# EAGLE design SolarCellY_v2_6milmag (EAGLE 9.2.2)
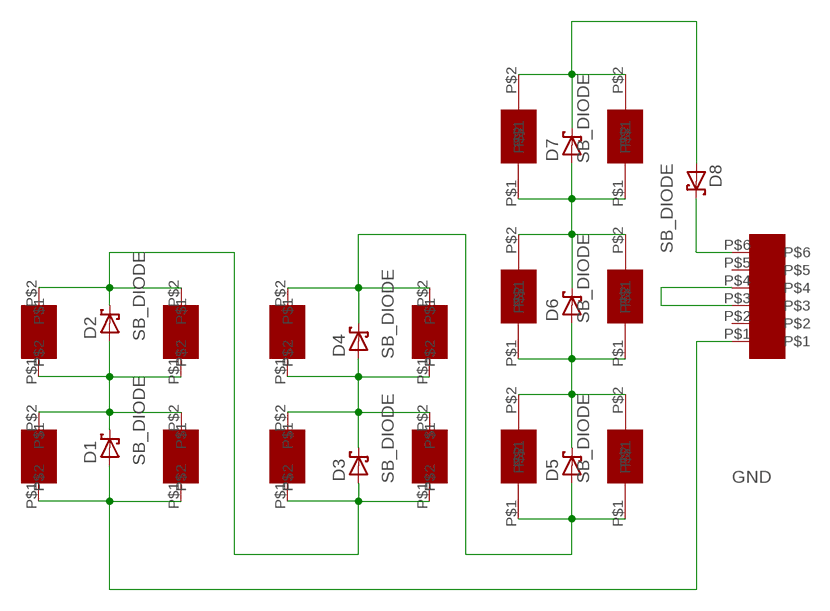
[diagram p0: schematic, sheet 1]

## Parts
11  SLMD121H04L  [SLMD121H04L]
12  SLMD121H04L  [SLMD121H04L]
13  SLMD121H04L  [SLMD121H04L]
14  SLMD121H04L  [SLMD121H04L]
21  SLMD121H04L  [SLMD121H04L]
22  SLMD121H04L  [SLMD121H04L]
23  SLMD121H04L  [SLMD121H04L]
24  SLMD121H04L  [SLMD121H04L]
D1  SB_DIODE  [SB_DIODE]
D2  SB_DIODE  [SB_DIODE]
D3  SB_DIODE  [SB_DIODE]
D4  SB_DIODE  [SB_DIODE]
D5  SB_DIODE  [SB_DIODE]
D6  SB_DIODE  [SB_DIODE]
D7  SB_DIODE  [SB_DIODE]
D8  SB_DIODE  [SB_DIODE]
U$1  M20-8760342  [M20-8760342]
U$2  KXOB22-04X3F  [KXOB22-04X3F]
U$3  KXOB22-04X3F  [KXOB22-04X3F]
U$4  KXOB22-04X3F  [KXOB22-04X3F]
U$5  KXOB22-04X3F  [KXOB22-04X3F]
U$6  KXOB22-04X3F  [KXOB22-04X3F]
U$7  KXOB22-04X3F  [KXOB22-04X3F]

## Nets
GND: 11.P$1 12.P$1 D1.POS U$1.P$1
N$1: U$1.P$3 U$1.P$4
N$2: 11.P$2 12.P$2 13.P$1 14.P$1 D1.NEG D2.POS
N$3: 13.P$2 14.P$2 21.P$1 22.P$1 D2.NEG D3.POS
N$4: 23.P$2 24.P$2 D4.NEG D5.POS U$2.P$1 U$3.P$1
N$5: 21.P$2 22.P$2 23.P$1 24.P$1 D3.NEG D4.POS
N$6: D5.NEG D6.POS U$2.P$2 U$3.P$2 U$4.P$1 U$5.P$1
N$8: D6.NEG D7.POS U$4.P$2 U$5.P$2 U$6.P$1 U$7.P$1
N$10: D7.NEG D8.POS U$6.P$2 U$7.P$2
N$14: D8.NEG U$1.P$6
Unconnected: U$1.P$2 U$1.P$5

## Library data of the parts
11-14 21-24 = Solar:SLMD121H04L
D1-D8 = Solar:SB_DIODE
U$1 = Solar:M20-8760342
U$2-U$7 = Solar:KXOB22-04X3F

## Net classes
1 power: width 0.254 mm

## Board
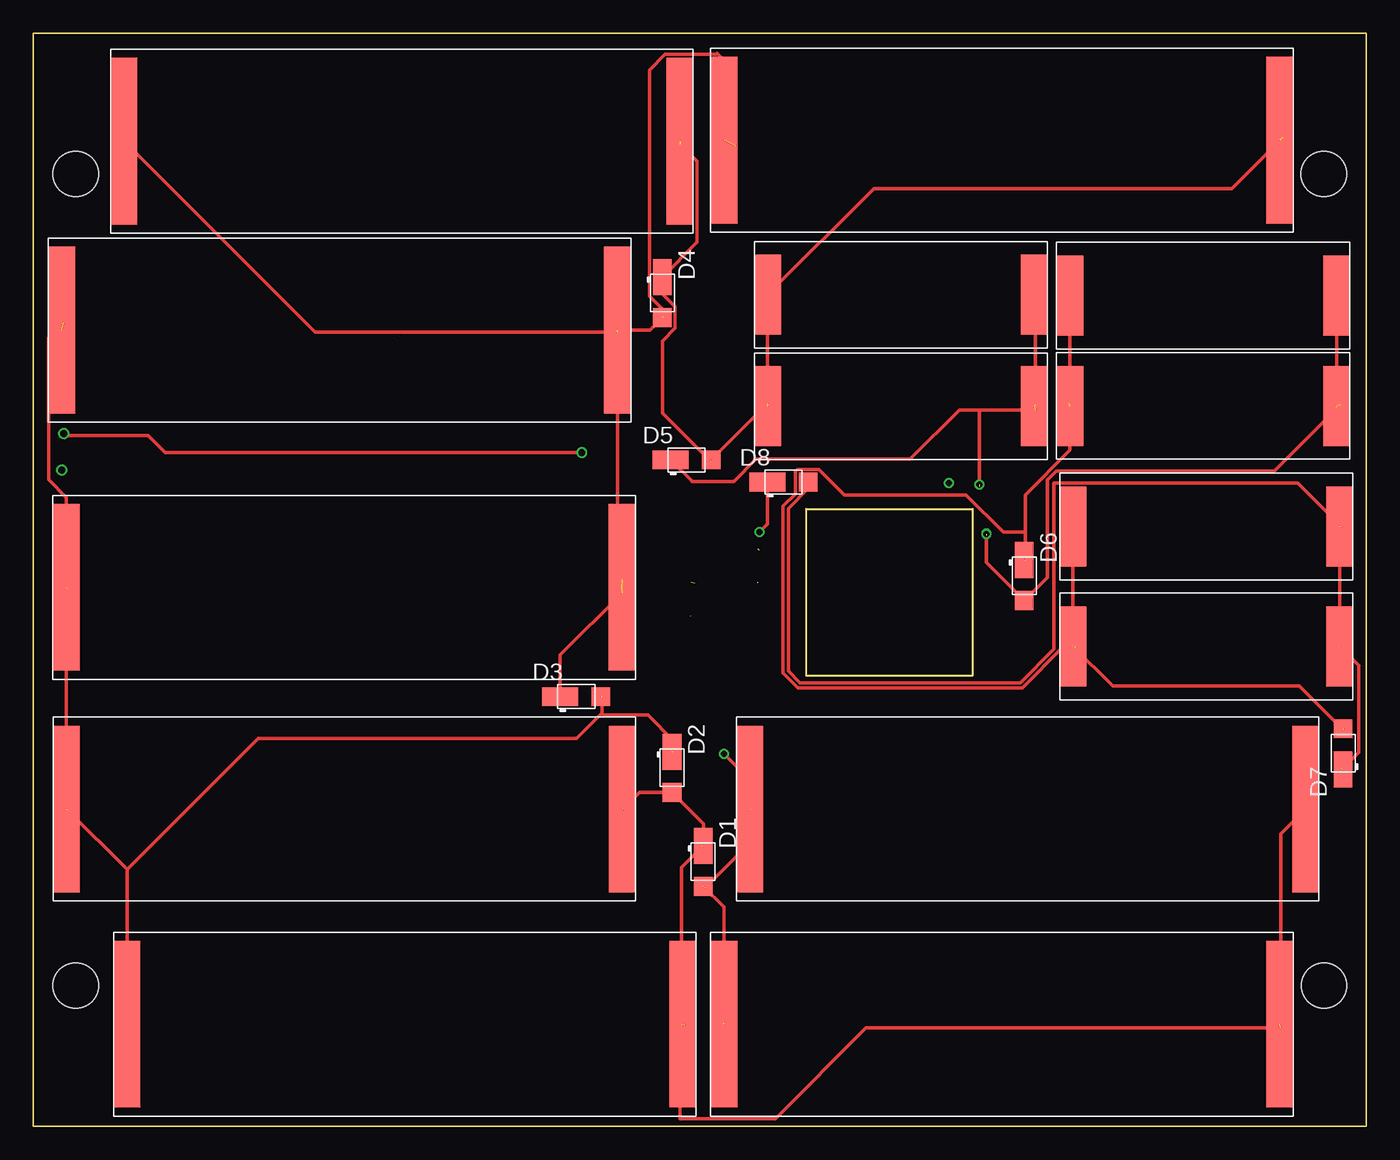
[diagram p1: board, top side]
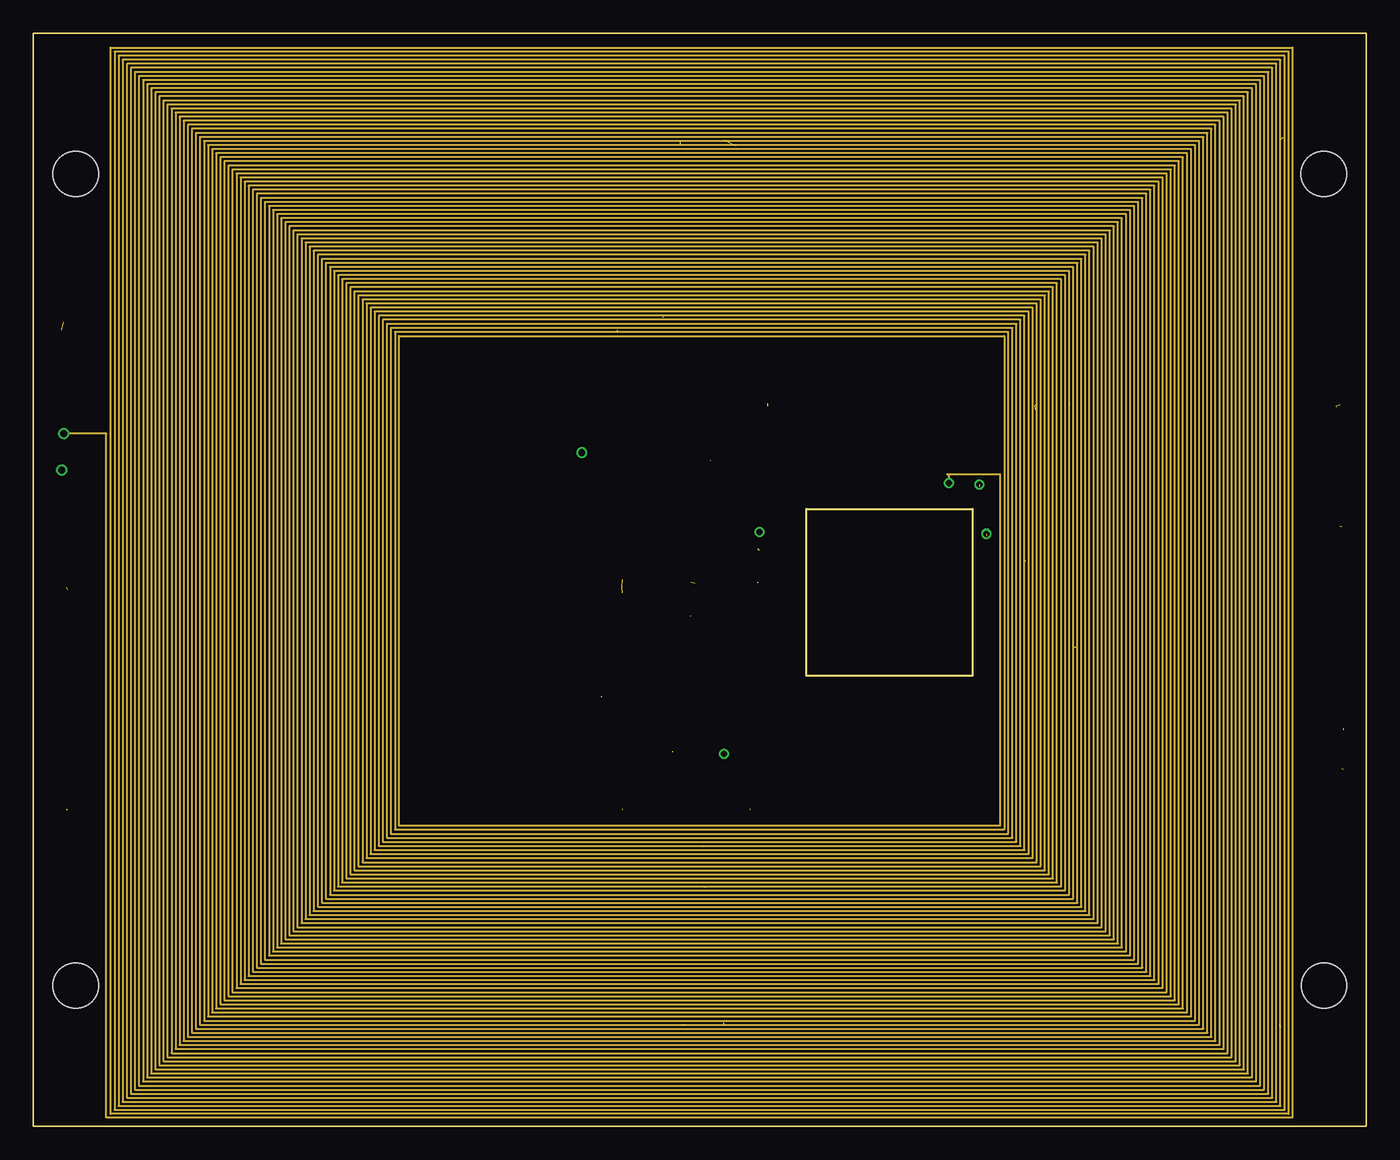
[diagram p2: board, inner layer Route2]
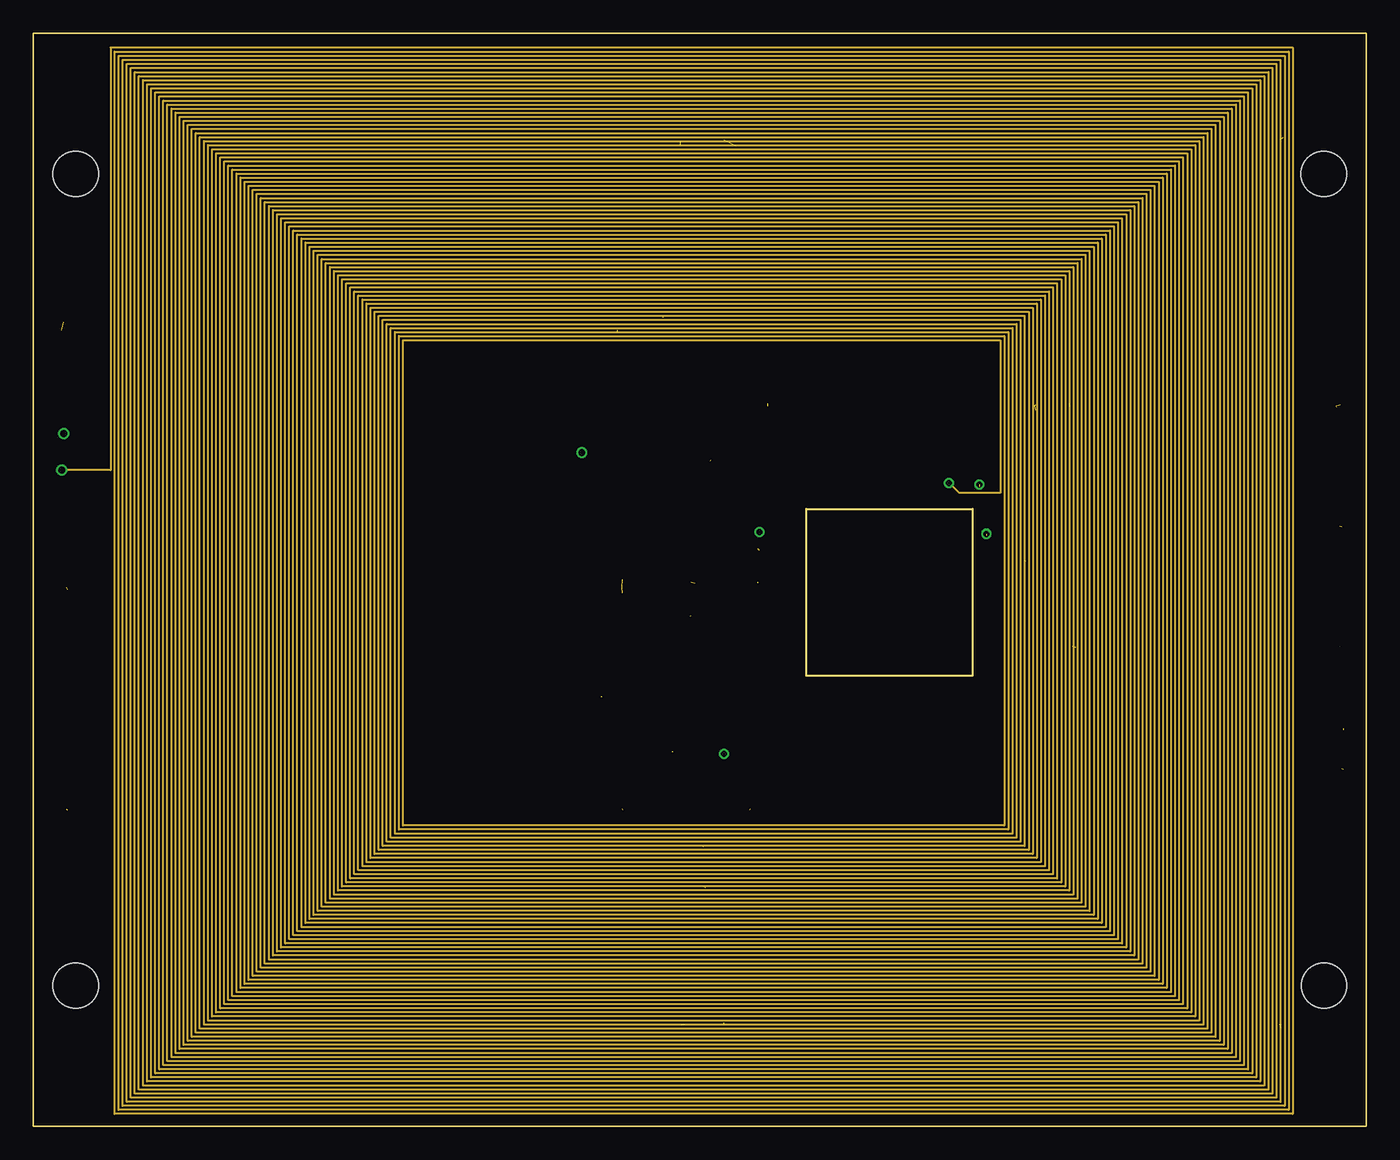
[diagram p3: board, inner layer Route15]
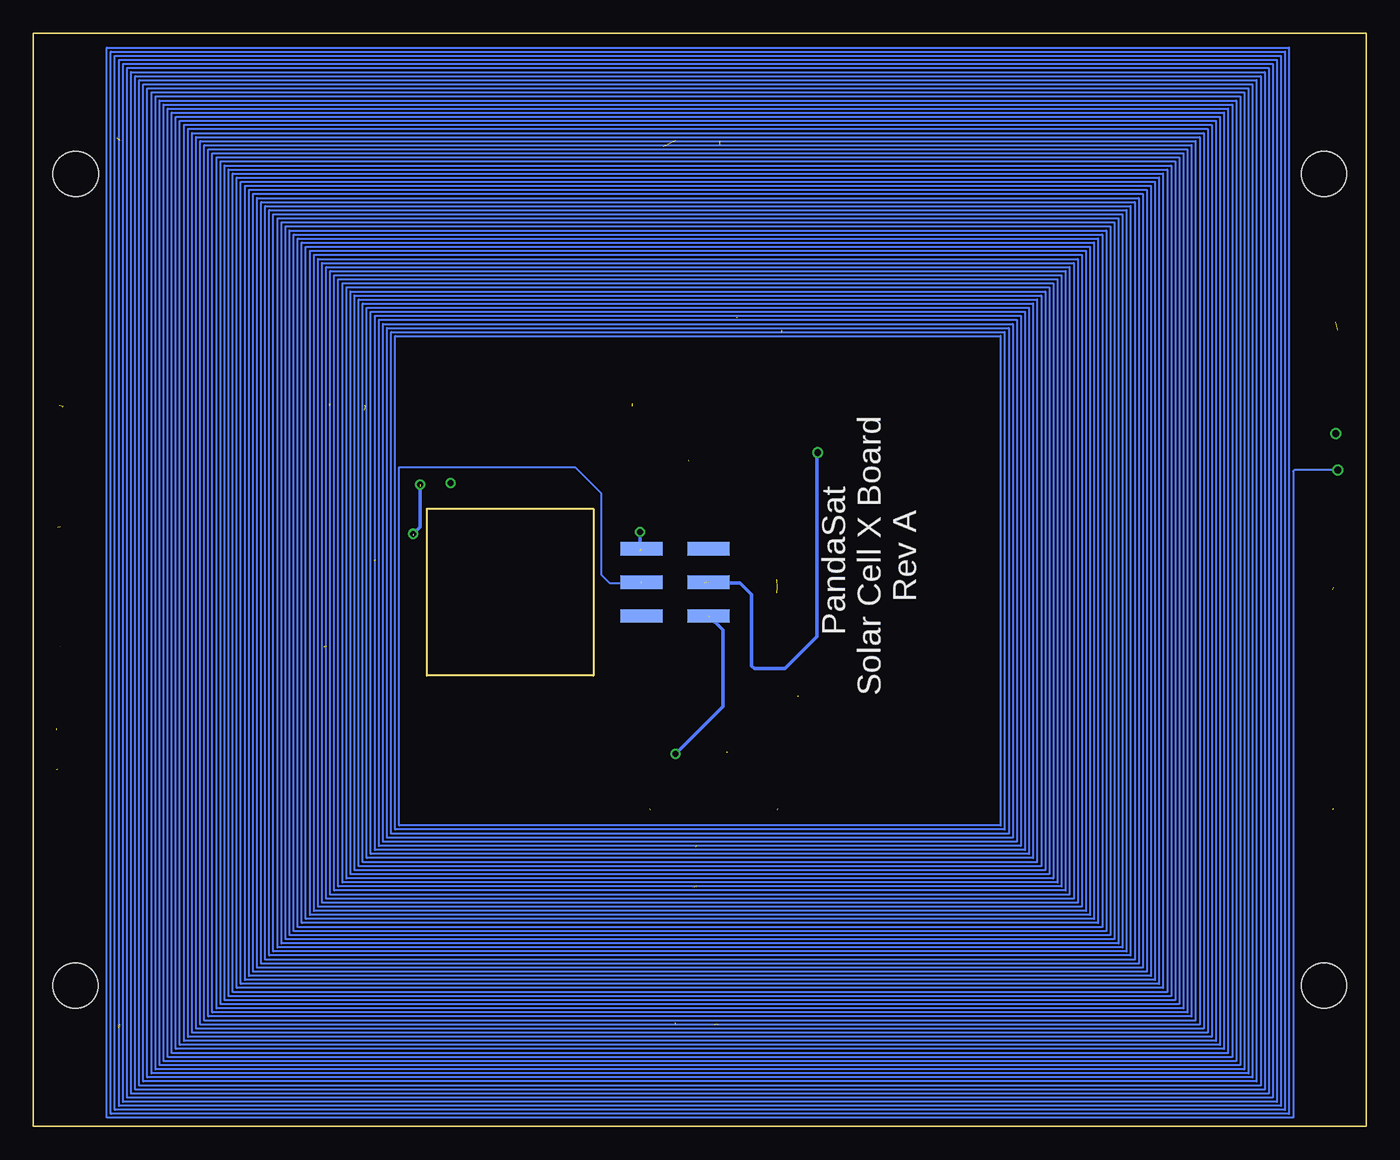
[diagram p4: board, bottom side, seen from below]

Size 100 x 82 mm. Coordinates in mm from the lower left corner, seen from the top.
Outline: 0,0 0,82 100,82 100,0 0,0
Copper layers (1*2*15*16): Top 0.035559375mm / dielectric 0.17018125mm / Route2 0.01778125mm / dielectric 47mil / Route15 0.01778125mm / dielectric 0.17018125mm / Bottom 0.035559375mm
Design rules "oshpark-4layer *": minimum track width 5mil, minimum drill 10mil, track to track 5mil, track to pad 5mil, pad to pad 5mil, via to via 5mil, smd to smd 5mil, copper to edge 15mil, drill to drill 6mil, minimum pad ring 4mil, minimum via ring 6mil, stop-mask expansion 2.5mil, vias tented up to drill 0mil, thermal gap 10mil
Holes 3.4 mm at 3.17,10.55 96.82,71.45 3.17,71.45 96.83,10.55
Milling: 4 lines

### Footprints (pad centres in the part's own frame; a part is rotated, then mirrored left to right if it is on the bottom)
SLMD121H04L = smd 2 x 12.5: P$1 1,6.9; P$2 42.7,6.9
SB_DIODE = smd 2.7 x 1.4: NEG -1.2,0 | smd 1.4 x 1.4: POS 1.85,0
M20-8760342 = smd 1 x 3.15: P$1 0.5,1.575; P$2 0.5,6.625; P$3 3.04,1.575; P$4 3.04,6.625; P$5 5.54,1.575; P$6 5.54,6.625
KXOB22-04X3F = smd 2 x 6: P$1 1,4; P$2 21,4

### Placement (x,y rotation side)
11  50.81,0.76 0 top
12  52.76,16.89 0 top
13  49.73,14.56 180 top
14  45.18,30.7 180 top
21  1.47,33.53 0 top
22  1.14,52.83 0 top
23  5.81,67.01 0 top
24  50.81,67.08 0 top
D1  50.26,19.85 270 top
D2  47.92,26.9 270 top
D3  40.73,32.23 0 top
D4  47.19,62.52 270 top
D5  49,50 0 top
D6  74.35,41.3 270 top
D7  98.27,27.98 90 top
D8  56.28,48.33 0 top
U$1  47.75,37.78 90 bottom
U$2  54.09,58.38 0 top
U$3  54.09,50.02 0 top
U$4  98.77,66.31 180 top
U$5  98.77,58.04 180 top
U$6  77,41 0 top
U$7  77,32 0 top

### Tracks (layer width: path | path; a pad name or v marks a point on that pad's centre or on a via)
GND  (via drill 0.45)  (4 unrouted)
  Top 0.254: v51.82,27.94 53.72,26.04 53.72,23.75 | 12.P$1 53.76,21.24 50.42,17.91 | D1.POS 51.82,16.44 51.82,7.75
  Bottom 0.152: 49.28,38.41 49.28,38.35 | 49.28,38.23 49.28,38.35 | 49.28,38.35 48.77,38.35
  Bottom 0.254: U$1.P$1 48.26,37.22 48.26,31.5 v51.82,27.94
N$1  (via drill 0.45, 0.5)  (3 unrouted)
  Top 0.254: v41.15,50.55 9.91,50.55 8.64,51.82 2.41,51.82 2.29,51.94 v2.29,51.97
  Route2 0.152: v2.29,51.97 5.49,51.97 5.49,0.65 94.49,0.65 94.49,80.92 5.79,80.92 5.79,0.91 94.18,0.91 94.18,80.62 6.1,80.62 6.1,1.22 93.88,1.22 93.88,80.31 6.4,80.31 6.4,1.52 93.57,1.52 93.57,80.01 6.71,80.01 6.71,1.83 93.27,1.83 93.27,79.7 7.01,79.7 7.01,2.13 92.96,2.13 92.96,79.4 7.32,79.4 7.32,2.44 92.66,2.44 92.66,79.1 7.62,79.1 7.62,2.74 92.35,2.74 92.35,78.79 7.92,78.79 7.92,3.05 92.05,3.05 92.05,78.49 8.23,78.49 8.23,3.35 91.75,3.35 91.75,78.18 8.53,78.18 8.53,3.66 91.44,3.66 91.44,77.88 8.84,77.88 8.84,3.96 91.14,3.96 91.14,77.57 9.14,77.57 9.14,4.27 90.83,4.27 90.83,77.27 9.45,77.27 9.45,4.57 90.53,4.57 90.53,76.96 9.75,76.96 9.75,4.88 90.22,4.88 90.22,76.66 10.06,76.66 10.06,5.18 89.92,5.18 89.92,76.35 10.36,76.35 10.36,5.49 89.61,5.49 89.61,76.05 10.67,76.05 10.67,5.79 89.31,5.79 89.31,75.74 10.97,75.74 10.97,6.1 89,6.1 89,75.44 11.28,75.44 11.28,6.4 88.7,6.4 88.7,75.13 11.58,75.13 11.58,6.71 88.39,6.71 88.39,74.83 11.89,74.83 11.89,7.01 88.09,7.01 88.09,74.52 12.19,74.52 12.19,7.32 87.78,7.32 87.78,74.22 12.5,74.22 12.5,7.62 87.48,7.62 87.48,73.91 12.8,73.91 12.8,7.92 87.17,7.92 87.17,73.61 13.11,73.61 13.11,8.23 86.87,8.23 86.87,73.3 13.41,73.3 13.41,8.53 86.56,8.53 86.56,73 13.72,73 13.72,8.84 86.26,8.84 86.26,72.69 14.02,72.69 14.02,9.14 85.95,9.14 85.95,72.39 14.33,72.39 14.33,9.45 85.65,9.45 85.65,72.08 14.63,72.08 14.63,9.75 85.34,9.75 85.34,71.78 14.94,71.78 14.94,10.06 85.04,10.06 85.04,71.48 15.24,71.48 15.24,10.36 84.73,10.36 84.73,71.17 15.54,71.17 15.54,10.67 84.43,10.67 84.43,70.87 15.85,70.87 15.85,10.97 84.12,10.97 84.12,70.56 16.15,70.56 16.15,11.28 83.82,11.28 83.82,70.26 16.46,70.26 16.46,11.58 83.52,11.58 83.52,69.95 16.76,69.95 16.76,11.89 83.21,11.89 83.21,69.65 17.07,69.65 17.07,12.19 82.91,12.19 82.91,69.34 17.37,69.34 17.37,12.5 82.6,12.5 82.6,69.04 17.68,69.04 17.68,12.8 82.3,12.8 82.3,68.73 17.98,68.73 17.98,13.11 81.99,13.11 81.99,68.43 18.29,68.43 18.29,13.41 81.69,13.41 81.69,68.12 18.59,68.12 18.59,13.72 81.38,13.72 81.38,67.82 18.9,67.82 18.9,14.02 81.08,14.02 81.08,67.51 19.2,67.51 19.2,14.33 80.77,14.33 80.77,67.21 19.51,67.21 19.51,14.63 80.47,14.63 80.47,66.9 19.81,66.9 19.81,14.94 80.16,14.94 80.16,66.6 20.12,66.6 20.12,15.24 79.86,15.24 79.86,66.29 20.42,66.29 20.42,15.54 79.55,15.54 79.55,65.99 20.73,65.99 20.73,15.85 79.25,15.85 79.25,65.68 21.03,65.68 21.03,16.15 78.94,16.15 78.94,65.38 21.34,65.38 21.34,16.46 78.64,16.46 78.64,65.08 21.64,65.08 21.64,16.76 78.33,16.76 78.33,64.77 21.95,64.77 21.95,17.07 78.03,17.07 78.03,64.47 22.25,64.47 22.25,17.37 77.72,17.37 77.72,64.16 22.55,64.16 22.55,17.68 77.42,17.68 77.42,63.86 22.86,63.86 22.86,17.98 77.11,17.98 77.11,63.55 23.16,63.55 23.16,18.29 76.81,18.29 76.81,63.25 23.47,63.25 23.47,18.59 76.5,18.59 76.5,62.94 23.77,62.94 23.77,18.9 76.2,18.9 76.2,62.64 24.08,62.64 24.08,19.2 75.89,19.2 75.89,62.33 24.38,62.33 24.38,19.51 75.59,19.51 75.59,62.03 24.69,62.03 24.69,19.81 75.29,19.81 75.29,61.72 24.99,61.72 24.99,20.12 74.98,20.12 74.98,61.42 25.3,61.42 25.3,20.42 74.68,20.42 74.68,61.11 25.6,61.11 25.6,20.73 74.37,20.73 74.37,60.81 25.91,60.81 25.91,21.03 74.07,21.03 74.07,60.5 26.21,60.5 26.21,21.34 73.76,21.34 73.76,60.2 26.52,60.2 26.52,21.64 73.46,21.64 73.46,59.89 26.82,59.89 26.82,21.95 73.15,21.95 73.15,59.59 27.13,59.59 27.13,22.25 72.85,22.25 72.85,59.28 27.43,59.28 27.43,22.55 72.54,22.55 72.54,48.9 68.58,48.9 68.71,48.77 v68.71,48.26
  Route15 0.152: v2.13,49.23 5.79,49.23 5.79,80.92 94.49,80.92 94.49,0.91 6.1,0.91 6.1,80.62 94.18,80.62 94.18,1.22 6.4,1.22 6.4,80.31 93.88,80.31 93.88,1.52 6.71,1.52 6.71,80.01 93.57,80.01 93.57,1.83 7.01,1.83 7.01,79.7 93.27,79.7 93.27,2.13 7.32,2.13 7.32,79.4 92.96,79.4 92.96,2.44 7.62,2.44 7.62,79.1 92.66,79.1 92.66,2.74 7.92,2.74 7.92,78.79 92.35,78.79 92.35,3.05 8.23,3.05 8.23,78.49 92.05,78.49 92.05,3.35 8.53,3.35 8.53,78.18 91.75,78.18 91.75,3.66 8.84,3.66 8.84,77.88 91.44,77.88 91.44,3.96 9.14,3.96 9.14,77.57 91.14,77.57 91.14,4.27 9.45,4.27 9.45,77.27 90.83,77.27 90.83,4.57 9.75,4.57 9.75,76.96 90.53,76.96 90.53,4.88 10.06,4.88 10.06,76.66 90.22,76.66 90.22,5.18 10.36,5.18 10.36,76.35 89.92,76.35 89.92,5.49 10.67,5.49 10.67,76.05 89.61,76.05 89.61,5.79 10.97,5.79 10.97,75.74 89.31,75.74 89.31,6.1 11.28,6.1 11.28,75.44 89,75.44 89,6.4 11.58,6.4 11.58,75.13 88.7,75.13 88.7,6.71 11.89,6.71 11.89,74.83 88.39,74.83 88.39,7.01 12.19,7.01 12.19,74.52 88.09,74.52 88.09,7.32 12.5,7.32 12.5,74.22 87.78,74.22 87.78,7.62 12.8,7.62 12.8,73.91 87.48,73.91 87.48,7.92 13.11,7.92 13.11,73.61 87.17,73.61 87.17,8.23 13.41,8.23 13.41,73.3 86.87,73.3 86.87,8.53 13.72,8.53 13.72,73 86.56,73 86.56,8.84 14.02,8.84 14.02,72.69 86.26,72.69 86.26,9.14 14.33,9.14 14.33,72.39 85.95,72.39 85.95,9.45 14.63,9.45 14.63,72.08 85.65,72.08 85.65,9.75 14.94,9.75 14.94,71.78 85.34,71.78 85.34,10.06 15.24,10.06 15.24,71.48 85.04,71.48 85.04,10.36 15.54,10.36 15.54,71.17 84.73,71.17 84.73,10.67 15.85,10.67 15.85,70.87 84.43,70.87 84.43,10.97 16.15,10.97 16.15,70.56 84.12,70.56 84.12,11.28 16.46,11.28 16.46,70.26 83.82,70.26 83.82,11.58 16.76,11.58 16.76,69.95 83.52,69.95 83.52,11.89 17.07,11.89 17.07,69.65 83.21,69.65 83.21,12.19 17.37,12.19 17.37,69.34 82.91,69.34 82.91,12.5 17.68,12.5 17.68,69.04 82.6,69.04 82.6,12.8 17.98,12.8 17.98,68.73 82.3,68.73 82.3,13.11 18.29,13.11 18.29,68.43 81.99,68.43 81.99,13.41 18.59,13.41 18.59,68.12 81.69,68.12 81.69,13.72 18.9,13.72 18.9,67.82 81.38,67.82 81.38,14.02 19.2,14.02 19.2,67.51 81.08,67.51 81.08,14.33 19.51,14.33 19.51,67.21 80.77,67.21 80.77,14.63 19.81,14.63 19.81,66.9 80.47,66.9 80.47,14.94 20.12,14.94 20.12,66.6 80.16,66.6 80.16,15.24 20.42,15.24 20.42,66.29 79.86,66.29 79.86,15.54 20.73,15.54 20.73,65.99 79.55,65.99 79.55,15.85 21.03,15.85 21.03,65.68 79.25,65.68 79.25,16.15 21.34,16.15 21.34,65.38 78.94,65.38 78.94,16.46 21.64,16.46 21.64,65.08 78.64,65.08 78.64,16.76 21.95,16.76 21.95,64.77 78.33,64.77 78.33,17.07 22.25,17.07 22.25,64.47 78.03,64.47 78.03,17.37 22.55,17.37 22.55,64.16 77.72,64.16 77.72,17.68 22.86,17.68 22.86,63.86 77.42,63.86 77.42,17.98 23.16,17.98 23.16,63.55 77.11,63.55 77.11,18.29 23.47,18.29 23.47,63.25 76.81,63.25 76.81,18.59 23.77,18.59 23.77,62.94 76.5,62.94 76.5,18.9 24.08,18.9 24.08,62.64 76.2,62.64 76.2,19.2 24.38,19.2 24.38,62.33 75.89,62.33 75.89,19.51 24.69,19.51 24.69,62.03 75.59,62.03 75.59,19.81 24.99,19.81 24.99,61.72 75.29,61.72 75.29,20.12 25.3,20.12 25.3,61.42 74.98,61.42 74.98,20.42 25.6,20.42 25.6,61.11 74.68,61.11 74.68,20.73 25.91,20.73 25.91,60.81 74.37,60.81 74.37,21.03 26.21,21.03 26.21,60.5 74.07,60.5 74.07,21.34 26.52,21.34 26.52,60.2 73.76,60.2 73.76,21.64 26.82,21.64 26.82,59.89 73.46,59.89 73.46,21.95 27.13,21.95 27.13,59.59 73.15,59.59 73.15,22.25 27.43,22.25 27.43,59.28 72.85,59.28 72.85,22.55 27.74,22.55 27.74,58.98 72.54,58.98 72.54,47.52 69.47,47.52 68.71,48.28
  Bottom 0.152: v2.13,49.23 5.41,49.23 5.49,49.15 5.49,0.65 94.49,0.65 94.49,80.92 5.79,80.92 5.79,0.91 94.18,0.91 94.18,80.62 6.1,80.62 6.1,1.22 93.88,1.22 93.88,80.31 6.4,80.31 6.4,1.52 93.57,1.52 93.57,80.01 6.71,80.01 6.71,1.83 93.27,1.83 93.27,79.7 7.01,79.7 7.01,2.13 92.96,2.13 92.96,79.4 7.32,79.4 7.32,2.44 92.66,2.44 92.66,79.1 7.62,79.1 7.62,2.74 92.35,2.74 92.35,78.79 7.92,78.79 7.92,3.05 92.05,3.05 92.05,78.49 8.23,78.49 8.23,3.35 91.75,3.35 91.75,78.18 8.53,78.18 8.53,3.66 91.44,3.66 91.44,77.88 8.84,77.88 8.84,3.96 91.14,3.96 91.14,77.57 9.14,77.57 9.14,4.27 90.83,4.27 90.83,77.27 9.45,77.27 9.45,4.57 90.53,4.57 90.53,76.96 9.75,76.96 9.75,4.88 90.22,4.88 90.22,76.66 10.06,76.66 10.06,5.18 89.92,5.18 89.92,76.35 10.36,76.35 10.36,5.49 89.61,5.49 89.61,76.05 10.67,76.05 10.67,5.79 89.31,5.79 89.31,75.74 10.97,75.74 10.97,6.1 89,6.1 89,75.44 11.28,75.44 11.28,6.4 88.7,6.4 88.7,75.13 11.58,75.13 11.58,6.71 88.39,6.71 88.39,74.83 11.89,74.83 11.89,7.01 88.09,7.01 88.09,74.52 12.19,74.52 12.19,7.32 87.78,7.32 87.78,74.22 12.5,74.22 12.5,7.62 87.48,7.62 87.48,73.91 12.8,73.91 12.8,7.92 87.17,7.92 87.17,73.61 13.11,73.61 13.11,8.23 86.87,8.23 86.87,73.3 13.41,73.3 13.41,8.53 86.56,8.53 86.56,73 13.72,73 13.72,8.84 86.26,8.84 86.26,72.69 14.02,72.69 14.02,9.14 85.95,9.14 85.95,72.39 14.33,72.39 14.33,9.45 85.65,9.45 85.65,72.08 14.63,72.08 14.63,9.75 85.34,9.75 85.34,71.78 14.94,71.78 14.94,10.06 85.04,10.06 85.04,71.48 15.24,71.48 15.24,10.36 84.73,10.36 84.73,71.17 15.54,71.17 15.54,10.67 84.43,10.67 84.43,70.87 15.85,70.87 15.85,10.97 84.12,10.97 84.12,70.56 16.15,70.56 16.15,11.28 83.82,11.28 83.82,70.26 16.46,70.26 16.46,11.58 83.52,11.58 83.52,69.95 16.76,69.95 16.76,11.89 83.21,11.89 83.21,69.65 17.07,69.65 17.07,12.19 82.91,12.19 82.91,69.34 17.37,69.34 17.37,12.5 82.6,12.5 82.6,69.04 17.68,69.04 17.68,12.8 82.3,12.8 82.3,68.73 17.98,68.73 17.98,13.11 81.99,13.11 81.99,68.43 18.29,68.43 18.29,13.41 81.69,13.41 81.69,68.12 18.59,68.12 18.59,13.72 81.38,13.72 81.38,67.82 18.9,67.82 18.9,14.02 81.08,14.02 81.08,67.51 19.2,67.51 19.2,14.33 80.77,14.33 80.77,67.21 19.51,67.21 19.51,14.63 80.47,14.63 80.47,66.9 19.81,66.9 19.81,14.94 80.16,14.94 80.16,66.6 20.12,66.6 20.12,15.24 79.86,15.24 79.86,66.29 20.42,66.29 20.42,15.54 79.55,15.54 79.55,65.99 20.73,65.99 20.73,15.85 79.25,15.85 79.25,65.68 21.03,65.68 21.03,16.15 78.94,16.15 78.94,65.38 21.34,65.38 21.34,16.46 78.64,16.46 78.64,65.08 21.64,65.08 21.64,16.76 78.33,16.76 78.33,64.77 21.95,64.77 21.95,17.07 78.03,17.07 78.03,64.47 22.25,64.47 22.25,17.37 77.72,17.37 77.72,64.16 22.55,64.16 22.55,17.68 77.42,17.68 77.42,63.86 22.86,63.86 22.86,17.98 77.11,17.98 77.11,63.55 23.16,63.55 23.16,18.29 76.81,18.29 76.81,63.25 23.47,63.25 23.47,18.59 76.5,18.59 76.5,62.94 23.77,62.94 23.77,18.9 76.2,18.9 76.2,62.64 24.08,62.64 24.08,19.2 75.89,19.2 75.89,62.33 24.38,62.33 24.38,19.51 75.59,19.51 75.59,62.03 24.69,62.03 24.69,19.81 75.29,19.81 75.29,61.72 24.99,61.72 24.99,20.12 74.98,20.12 74.98,61.42 25.3,61.42 25.3,20.42 74.68,20.42 74.68,61.11 25.6,61.11 25.6,20.73 74.37,20.73 74.37,60.81 25.91,60.81 25.91,21.03 74.07,21.03 74.07,60.5 26.21,60.5 26.21,21.34 73.76,21.34 73.76,60.2 26.52,60.2 26.52,21.64 73.46,21.64 73.46,59.89 26.82,59.89 26.82,21.95 73.15,21.95 73.15,59.59 27.13,59.59 27.13,22.25 72.85,22.25 72.85,59.28 27.43,59.28 27.43,22.55 72.54,22.55 72.54,49.45 59.36,49.45 57.4,47.5 57.4,41.4 56.77,40.77 54.36,40.77
  Bottom 0.254: v41.15,50.55 41.2,50.55 41.2,36.75 43.62,34.33 45.88,34.33 46.1,34.54 46.1,39.88 46.99,40.77 49.66,40.77
N$2  (5 unrouted)
  Top 0.254: 44.2,23.75 45.5,25.05 D2.POS 50.29,22.68 50.29,20.95 | D1.NEG 48.64,19.43 48.64,7.62 | 12.P$2 93.6,21.94 93.6,7.37 62.48,7.37 55.69,0.57 48.51,0.57 48.51,7.24 48.9,7.62
N$3  (5 unrouted)
  Top 0.254: 13.P$2 7.03,19.26 | 7.03,19.26 2.54,23.75 | 7.03,19.26 16.86,29.08 40.77,29.08 42.67,30.99 | 42.67,30.99 42.67,32.26 | 42.67,30.99 42.8,30.86 46.1,30.86 48.01,28.96 48.01,28.07 | 14.P$2 2.48,40.2 2.54,40.26 | 21.P$1 2.47,47.19 1.14,48.51 1.14,59.18 2.29,60.33
N$4  (4 unrouted)
  Top 0.254: 50.8,49.91 47.19,53.52 47.19,58.91 48.14,59.87 48.14,61.48 47.19,62.43 D4.NEG 49.78,66.32 49.78,72.39 48.51,73.66 | D5.POS 55.08,54.23 55.24,54.23 | U$3.P$1 U$2.P$1 63.07,70.36 89.92,70.36 93.73,74.17
N$5  (5 unrouted)
  Top 0.254: D3.NEG 39.53,35.34 44.2,40.01 | 23.P$1 21.16,59.56 43.81,59.56 | 44.2,41.02 43.84,41.38 22.P$2 46.27,59.73 47.24,60.71 | D4.POS 47.19,61.31 46.24,62.27 46.24,79.25 47.4,80.42 51.2,80.42 51.31,80.52 52.7,79.12 52.7,73.53
N$6  (via drill 0.45)  (6 unrouted)
  Top 0.254: U$2.P$2 75.18,62.29 75.18,54.1 | 97.19,61.74 U$4.P$1 97.79,62.29 97.79,53.98 | 98.04,54.1 93.09,49.15 76.74,49.15 76.07,48.48 76.07,41.17 D6.POS 71.5,42.29 71.5,44.32 | D5.NEG 49.4,48.4 49.4,48.39 52.58,48.39 54.23,50.04 65.79,50.04 69.47,53.72 70.99,53.72 | 70.99,53.72 75.18,53.72 | v70.99,48.13 70.99,53.72
  Bottom 0.254: v71.5,44.45 70.99,44.96 70.99,48.01
N$8  (5 unrouted)
  Top 0.254: U$4.P$2 77.77,54.27 77.72,54.23 | U$5.P$2 77.77,50.71 74.42,47.37 74.42,44.58 | 74.42,44.58 74.42,42.42 | U$6.P$1 78,36.05 78.11,35.94 | U$7.P$1 80.98,33.02 95,33.02 98.3,29.72 | 78.23,35.94 77.25,35.94 74.2,32.89 57.37,32.89 56.26,34.01 56.26,46.51 57.18,47.43 57.18,49.14 57.33,49.29 58.94,49.29 60.86,47.37 69.98,47.37 72.77,44.58 74.42,44.58
N$10  (3 unrouted)
  Top 0.254: U$6.P$2 98,35.98 98.04,35.94 | U$7.P$2 99.43,34.57 99.43,28.05 98.17,26.8 | D8.POS 58.13,47.85 56.64,46.35 56.64,34.16 57.53,33.27 74.04,33.27 76.58,35.81 76.58,48.26 94.87,48.26 98.17,44.96
N$14  (via drill 0.45)  (1 unrouted)
  Top 0.254: D8.NEG 55.09,45.18 v54.48,44.58
  Bottom 0.254: v54.48,44.58 54.48,43.18

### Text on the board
bPlace: PandaSat / Solar Cell X Board / Rev A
